TYPE ConfigPM :
STRUCT
	//TurboN2FlowSetPoint:LREAL;			//0-200		mtorr
	TurboN2Pressure:INT;
	PrepareTransferTimeout:INT;				//1-99999	s
	TransferWaferTimeout:INT;				//1-99999	s
	OpenGasValveTimeout:INT;				//0-60		s
	CloseGasValveTimeout:INT;				//0-10
	OpenCloseSlitValveTimeout:INT;			//0-10
	GasFlowPressureAlarmRange:LREAL;		//0-760000	mtorr
	GasFlowPressureAlarmTime:LREAL;			//0-3600	s
	GasFlowPressureWarningRange:LREAL;		//0-760000	mtorr
	GasFlowPressureWarningTime:LREAL;		//0-3600	s
	EnableThrottleValve:BOOL;				//0-10				//不清楚作用
	ValveHeaterSetPointLimit:INT;			//0-500
	ForeLineHeaterSetPointLimit:INT;		//0-500
	CheckSubstrateTempTimeout:INT;			//0-3600			//不清楚作用
	CheckATMTimeout:INT;					//0-3000	s
	OverVentTime:UINT;						//0-60000	ms		充气至常压
	ChamberBasePressureThreshold:UDINT;		//0-1000000	mtorr	腔体基础压力门槛	工艺开始压力？腔体压力下限？
	ChamberBaseTemperatureThreshold:LREAL;	//0-1000	℃		腔体基础温度门槛	工艺开始温度？腔体温度下限？
	ProcessPressureOffset:LREAL;			//0-100		mtorr
	PickDelayTime:INT;						//0-10000	ms
	PlaceDelayTime:INT;						//0-10000	ms
	ChamberLabel:STRING;					//''
	WallHeaterSetPointLimit:INT;			//0-500
	PendulumHeaterSetPointLimit:INT;		//0-500
	EnableWallHeater:BOOL;					//0-10
	EnableGridHeater:BOOL;					//0-10
	(*RecipeToleranceIgnoreTime:INT;		//0-60		s	Tolerance失效时间,用不到*)
	RecipeRunningMode:INT;					//0-5
	ForelineInterlockPressure:LREAL;		//500-2000	℃
	IsEnableRecipeExtension:BOOL;			//0-10
	ControlPressureSetPoint:INT;			//0-2000	mtorr
	ControlPressureN2FlowSetPoint:INT;		//0-500		sccm	
	PMStableTime:INT;						//0-100		s
END_STRUCT
END_TYPE
